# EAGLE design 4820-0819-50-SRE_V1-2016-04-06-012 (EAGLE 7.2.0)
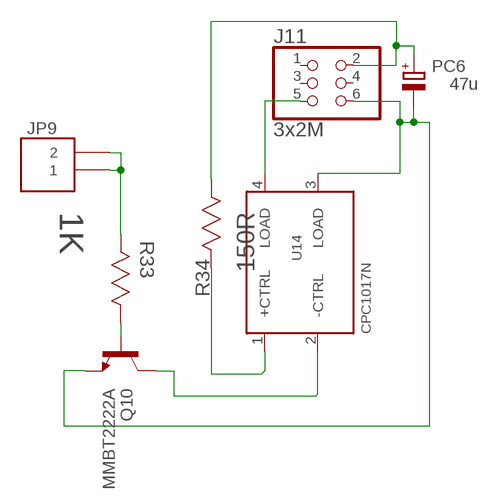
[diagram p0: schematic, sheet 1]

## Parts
J11  3x2M  PINHD-2X3  [2X03]
JP9  CONN_2PINCONN_2PIN_P2.54MM  [CONN_2PIN_P2.54MM]
PC6  47u  CPOL-EUD  [PANASONIC_D]
Q10  MMBT2222A  TRANSISTOR_NPNMMBT2222A  [SOT23-3]
R33  1K  CRM0805-FW-R050ELF  [RESC2013X65N]
R34  150R  CRM0805-FW-R050ELF  [RESC2013X65N]
U14  CPC1017N  CPC1125N  [SOP-4]

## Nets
N$1: J11.5 U14.4(LOAD)
N$3: J11.6 PC6.- Q10.2(E) U14.3(LOAD)
N$8: Q10.3(C) U14.2(-CTRL)
N$9: Q10.1(B) R33.1(R1)
N$12: R34.2(R2) U14.1(+CTRL)
N$13: J11.2 PC6.+ R34.1(R1)
N$46: JP9.1 JP9.2 R33.2(R2)
Unconnected: J11.1 J11.3 J11.4

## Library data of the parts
J11 = SmartPrj:PINHD-2X3: PIN HEADER
JP9 = VS_Eagle:CONN_2PIN
PC6 = rcl:CPOL-EU: POLARIZED CAPACITOR, European symbol
Q10 = SparkFun-DiscreteSemi:TRANSISTOR_NPN: Generic NPN BJT MMBT2222A - TRANS-08049 (SOT-23, 1A 40V) MPSA42 - TRANS-09116 (SOT-23, 500mA 300V) MMBT5088LT1G - TRANS-11160 (SOT-23, 50 mA 30V) BC547 - COM-08928 (TO-92 45V 100mA) (1.Collector 2.Base 3.Emitter) 2N3904 - COM-00521 (TO-92 40V 200mA) (1.Emitter 2.Base 3.Collector) P2N2222A -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; PROD_ID: TRANS-08049
R33 R34 = Bourns_By_element14_Batch_1:CRM0805-FW-R050ELF: Resistor 0805; MPN: CRM0805-FW-R050ELF; OC_FARNELL: 1865234; OC_NEWARK: 17T4231; SUPPLIER: BOURNS; TOLERANCE: ±1 %; VALUE: 0.05 Ohm; WATTAGE: 0.25 W
U14 = VS_Eagle:CPC1125N

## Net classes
0 default: width 0.254 mm, drill 0.61 mm, clearance 0.203 mm

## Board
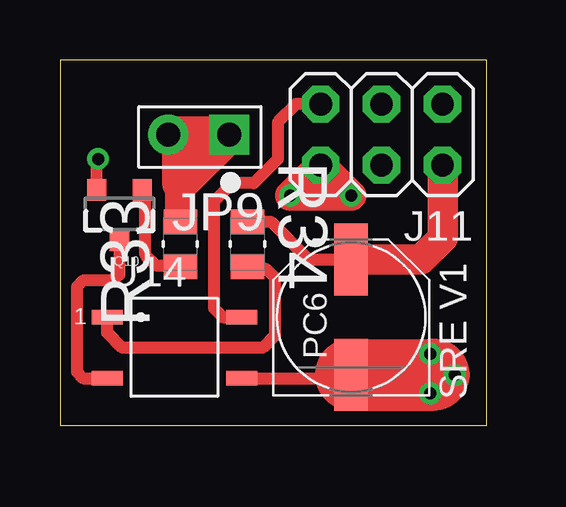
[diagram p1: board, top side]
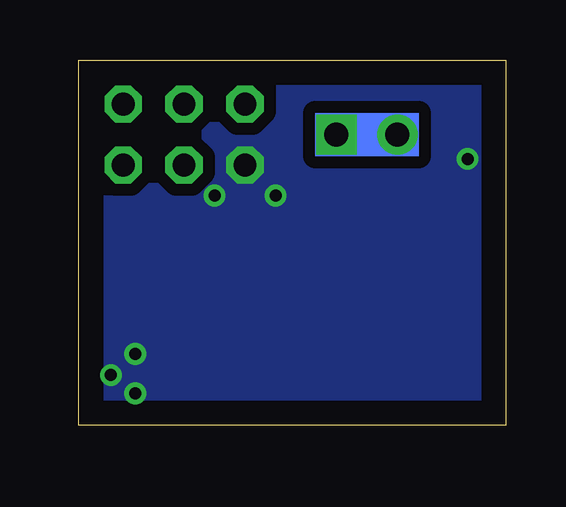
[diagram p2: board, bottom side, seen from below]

Size 17.78 x 15.24 mm. Coordinates in mm from the lower left corner, seen from the top.
Outline: 0,0 17.78,0 17.78,15.24 0,15.24 0,0
Copper layers (1*16): Top 0.035mm / dielectric 1.5mm / Bottom 0.035mm
Design rules "default": minimum track width 10mil, minimum drill 24mil, track to track 8mil, track to pad 8mil, pad to pad 8mil, via to via 8mil, smd to smd 8mil, copper to edge 40mil, drill to drill 8mil, minimum pad ring 10mil, minimum via ring 8mil, stop-mask expansion 4mil, vias tented up to drill 0mil, thermal gap 10mil

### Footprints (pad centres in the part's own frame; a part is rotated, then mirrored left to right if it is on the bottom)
2X03 = drill 0.95 pad 1.55 octagon: 1 -2.54,-1.27; 2 -2.54,1.27; 3 0,-1.27; 4 0,1.27; 5 2.54,-1.27; 6 2.54,1.27
CONN_2PIN_P2.54MM = drill 1 pad 1.676 square: 1 0,0 | drill 1 pad 1.676: 2 2.54,0
PANASONIC_D = smd 3 x 1.4: + 2.4,0; - -2.4,0
SOT23-3 = smd 0.8 x 0.9: 1 -0.95,-1; 2 0.95,-1; 3 0,1.1
RESC2013X65N = smd 1.016 x 1.397: 1 -0.94,0; 2 0.94,0
SOP-4 = smd 1.3 x 0.6: 1 0,0; 2 0,-2.54; 3 5.6,-2.54; 4 5.6,0

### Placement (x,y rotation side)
J11  13.4,12.13 180 top
JP9  7.05,12.13 180 top
PC6  12.13,4.51 90 top
Q10  2.48,8.83 180 top
R33  5.02,7.56 90 top
R34  7.81,7.56 270 top
U14  1.97,4.51 0 top

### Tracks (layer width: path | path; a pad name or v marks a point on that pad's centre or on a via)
N$1
  Top 0.508: J11.5 9.84,13.4 9.08,12.64 9.08,11.11 8.06,10.1 7.18,10.1 6.41,9.33 6.41,4.89 6.79,4.51 U14.4
N$3  (via drill 0.5)
  Top 0.508: U14.3 11.99,1.97 PC6.- | Q10.2 1.53,11.05 v1.59,11.11
  Top 1.27: v15.43,1.33 15.43,2.1 v15.43,2.98 v16.45,2.1 v15.43,1.33 | J11.6 v12.13,9.59 v9.59,9.59 J11.6
  Top 1.778: 15.57,2.11 15.43,2.1
  Top 2.997: PC6.- 15.57,2.11
  pour Bottom (isolate 0.508, no thermals): 0.7,0.7 16.95,0.7 16.95,14.41 0.7,14.41
N$8
  Top 0.508: Q10.3 2.48,6.29 2.22,6.03 0.95,6.03 0.7,5.78 0.7,2.22 0.95,1.97 U14.2
N$9
  Top 0.508: R33.1 4.97,6.67 4,6.67 3.55,7.11 3.55,9.7 Q10.1
N$12
  Top 0.508: R34.2 8.57,6.54 8.95,6.16 8.95,3.75 8.45,3.24 2.6,3.24 1.97,3.87 U14.1
N$13
  Top 0.508: R34.1 8.78,8.5 10.35,6.92 11.89,6.92 PC6.+
  Top 1.27: PC6.+ 15.04,6.91 15.94,7.81 J11.2
N$46
  Top 1.016: 5.02,8.95 R33.2
  Top 1.27: 5.02,8.95 5.02,10.1
  Top 1.524: JP9.2 5.02,12.13 | 5.02,12.13 JP9.1 5.02,10.1 5.02,12.13
(copper drawn outside any net)
  shapes: Bottom area x1

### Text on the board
tPlace: SRE V1

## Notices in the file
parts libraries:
SparkFun-DiscreteSemi: Licensing: Creative Commons ShareAlike 4.0 International - https://creativecommons.org/licenses/by-sa/4.0
